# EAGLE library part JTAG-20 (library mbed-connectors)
SUYIN Connector 20-pol
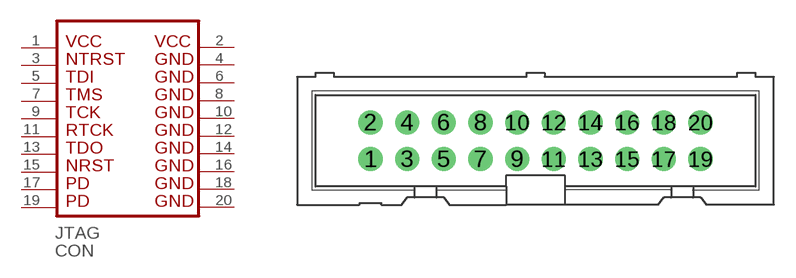
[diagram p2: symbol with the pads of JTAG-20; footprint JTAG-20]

Designator prefix CON

## JTAG-20  [JTAG-20]
1  1  pas
2  2  pas
3  3  pas
4  4  pas
5  5  pas
6  6  pas
7  7  pas
8  8  pas
9  9  pas
10  10  pas
11  11  pas
12  12  pas
13  13  pas
14  14  pas
15  15  pas
16  16  pas
17  17  pas
18  18  pas
19  19  pas
20  20  pas

## Footprint JTAG-20 (pad centres in mm)
SUYIN Connector 20-pol
drill 1.016 pad 1.676: 1 0,0; 2 0,2.54; 3 2.54,0; 4 2.54,2.54; 5 5.08,0; 6 5.08,2.54; 7 7.62,0; 8 7.62,2.54; 9 10.16,0; 10 10.16,2.54; 11 12.7,0; 12 12.7,2.54; 13 15.24,0; 14 15.24,2.54; 15 17.78,0; 16 17.78,2.54; 17 20.32,0; 18 20.32,2.54; 19 22.86,0; 20 22.86,2.54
